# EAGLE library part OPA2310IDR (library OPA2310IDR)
General Purpose Amplifier 2 Circuit Rail-to-Rail 8-SOIC Source: Datasheet
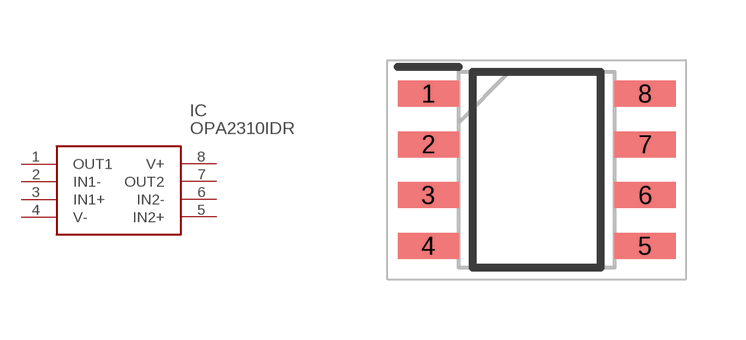
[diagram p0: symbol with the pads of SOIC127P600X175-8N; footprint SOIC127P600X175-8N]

Designator prefix IC

## OPA2310IDR (Description: General Purpose Amplifier 2 Circuit Rail-to-Rail 8-SOIC; Height: 1.75mm; Manufacturer_Name: Texas Instruments; Manufacturer_Part_Number: OPA2310IDR; Mouser_Part_Number: 595-OPA2310IDR; Mouser_Price-Stock: https://www.mouser.co.uk/ProductDetail/Texas-Instruments/OPA2310IDR?qs=vvQtp7zwQdO7M4WMfM7rQg%3D%3D)  [SOIC127P600X175-8N]
1  OUT1
2  IN1-
3  IN1+
4  V-
5  IN2+
6  IN2-
7  OUT2
8  V+

## Footprint SOIC127P600X175-8N (pad centres in mm)
(D0008A-H=1.75
smd 1.528 x 0.65: 1 -2.711,1.905; 2 -2.711,0.635; 3 -2.711,-0.635; 4 -2.711,-1.905; 5 2.711,-1.905; 6 2.711,-0.635; 7 2.711,0.635; 8 2.711,1.905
